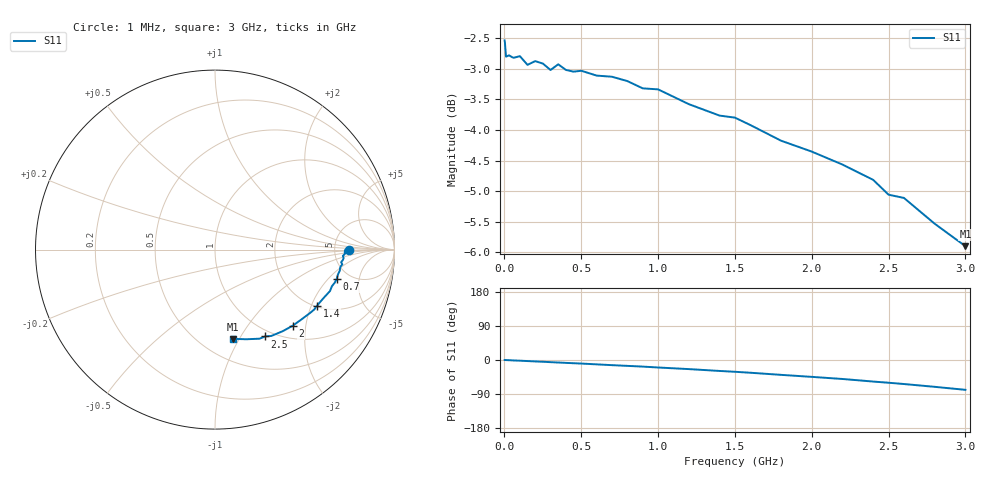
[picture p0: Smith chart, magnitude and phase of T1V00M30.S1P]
! SIEMENS Small Signal Semiconductors
! BAT68-04
! Si Schottky Diode (2 diodes in series, pin 3 open) in SOT23
! IF = 0.3 mA
! S-Parameters:  August  1994
# GHz  S  MA  R  50
!  f  S11
! GHz  MAG  ANG
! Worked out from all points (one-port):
!   33 points, 1 MHz to 3 GHz, reference 50 ohm
!   lowest |S11| = -5.9 dB at 3 GHz (marker M1), VSWR 3.06, Z = 35.1 - j47 ohm
!   |S11| at or under -10 dB: nowhere
!   S11 on the Smith chart (normalised r, x): 1 MHz: 6.90, +0.00; 700 MHz: 3.93, -2.51; 1.4 GHz: 2.03, -2.20; 2 GHz: 1.26, -1.69; 2.5 GHz: 0.91, -1.28; 3 GHz: 0.70, -0.94
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0.001  0.7468 0.0
0.003  0.7439 0.0
0.01  0.7243 -0.2
0.1  0.7251 -1.8
0.15  0.7133 -2.8
0.2  0.7183 -3.8
0.25  0.715 -4.6
0.3  0.7064 -5.7
0.35  0.714 -6.6
0.4  0.7065 -7.6
0.5  0.7054 -9.4
0.6  0.699 -11.5
0.7  0.6975 -13.6
0.8  0.6918 -15.5
0.9  0.6824 -17.4
1  0.6811 -19.8
1.2  0.6624 -24.0
1.4  0.6483 -28.9
1.5  0.6458 -31.1
1.6  0.6369 -33.6
1.8  0.6184 -39.2
2  0.6058 -44.5
2.2  0.5912 -50.1
2.4  0.5744 -56.9
2.5  0.5586 -60.0
2.6  0.5552 -63.4
2.8  0.5289 -70.8
3  0.507 -78.7
